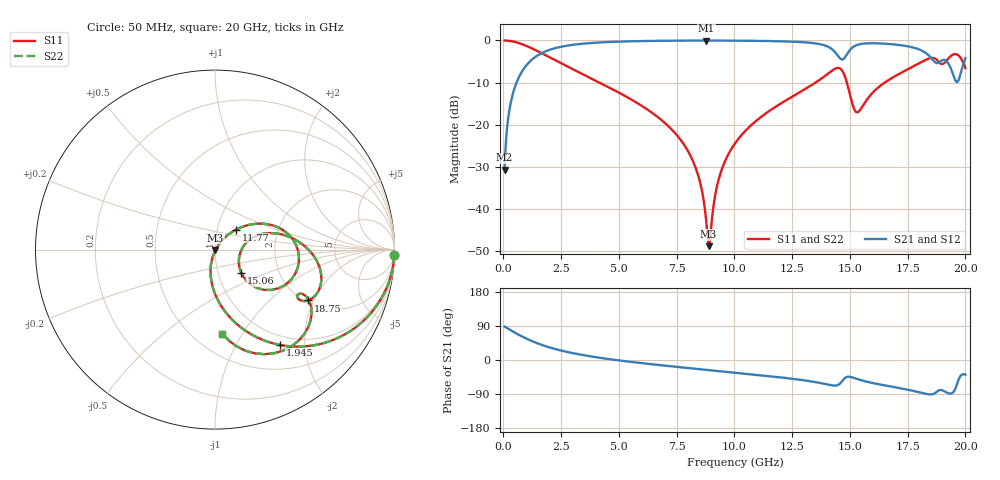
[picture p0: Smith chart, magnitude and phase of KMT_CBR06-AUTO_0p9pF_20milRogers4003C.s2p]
! Data measured by Modelithics Inc. support@modelithics.com 813-866-6335
! KEMET CBR06-AUTO 0.9pF, Pad Width= 0.851mm, Pad Length= 0.64mm, Pad Gap= 0.62mm, 20mil Rogers 4003C substrate Data, January 2022
# hz S ma R 50
! 2 Port Network Data from SP1.SP block
! freq  magS11  angS11  magS21  angS21  magS12  angS12  magS22  angS22
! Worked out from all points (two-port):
!   401 points, 50 MHz to 20 GHz, reference 50 ohm
!   highest |S21| = -0.03 dB at 8.778 GHz (marker M1); lowest = -30.6 dB at 50 MHz (marker M2)
!   |S21| within 3 dB of the highest: 1.649 GHz to 14.4 GHz (12.75 GHz wide, 159 % of centre); 14.9 GHz to 18.3 GHz (3.399 GHz wide, 20.5 % of centre)
!   lowest |S11| = -48.8 dB at 8.878 GHz (marker M3), VSWR 1.01, Z = 50.3 - j0.256 ohm
!   |S11| at or under -10 dB: 4.16 GHz to 13.51 GHz (9.351 GHz wide, 106 % of centre); 14.87 GHz to 16.51 GHz (1.637 GHz wide, 10.4 % of centre)
!   |S22| runs from -48.8 to 0.0 dB; largest |S21 - S12| = 0
!   S11 on the Smith chart (normalised r, x): 50 MHz: 1, -62; 1.945 GHz: 0.85, -1.54; 11.77 GHz: 1.23, +0.28; 15.06 GHz: 1.29, -0.35; 18.75 GHz: 2.09, -1.82; 20 GHz: 0.68, -0.82
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5e7  0.9996 -1.8  0.02938 88.2  0.02938 88.2  0.9996 -1.8
2.99375e8  0.9848 -10.9  0.1735 79.1  0.1735 79.1  0.9848 -10.9
5.98625e8  0.9427 -21.3  0.3329 68.7  0.3329 68.7  0.9427 -21.3
1.94525e9  0.6428 -55.7  0.7644 34.1  0.7644 34.1  0.6428 -55.7
3.391625e9  0.4032 -76.1  0.9129 13.6  0.9129 13.6  0.4032 -76.1
6.73325e9  0.1204 -101.9  0.9897 -13.3  0.9897 -13.3  0.1204 -101.9
8.179625e9  0.03852 -107.4  0.9957 -22.3  0.9957 -22.3  0.03852 -107.4
8.52875e9  0.01995 -104.7  0.9962 -24.4  0.9962 -24.4  0.01995 -104.7
8.778125e9  0.007266 -87.7  0.9962 -25.8  0.9962 -25.8  0.007266 -87.7
8.877875e9  0.003643 -44.3  0.9962 -26.4  0.9962 -26.4  0.003643 -44.3
9.376625e9  0.02559 52.3  0.9957 -29.4  0.9957 -29.4  0.02559 52.3
1.0025e10  0.06022 52.8  0.9938 -33.3  0.9938 -33.3  0.06022 52.8
1.177062e10  0.1627 43.4  0.9799 -44.3  0.9799 -44.3  0.1627 43.4
1.336662e10  0.2982 29.0  0.9329 -56.9  0.9329 -56.9  0.2982 29.0
1.451375e10  0.4718 -12.4  0.6397 -64.9  0.6397 -64.9  0.4718 -12.4
1.506238e10  0.1968 -41.7  0.803 -45.2  0.803 -45.2  0.1968 -41.7
1.536162e10  0.1421 -6.3  0.8935 -51.1  0.8935 -51.1  0.1421 -6.3
1.670825e10  0.3437 15.4  0.9067 -69.2  0.9067 -69.2  0.3437 15.4
1.875312e10  0.5921 -28.6  0.5384 -84.4  0.5384 -84.4  0.5921 -28.6
1.945138e10  0.6761 -39.8  0.4057 -86.4  0.4057 -86.4  0.6761 -39.8
1.965088e10  0.6792 -55.8  0.3211 -61.3  0.3211 -61.3  0.6792 -55.8
2e10  0.4705 -84.9  0.6143 -38.7  0.6143 -38.7  0.4705 -84.9
